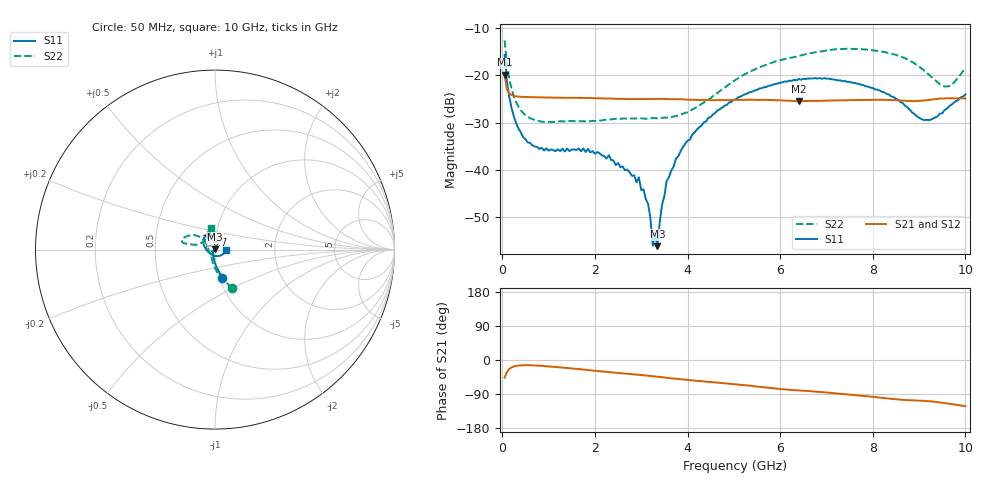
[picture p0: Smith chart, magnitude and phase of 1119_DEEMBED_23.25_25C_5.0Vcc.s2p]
!Hittite Microwave Corp.
!Digital Attenuator/PhaseShifter Rev 1.4.0
!Filename: C:\DATA\DATA\1119_DEEMBED_23.25_25C_5.0Vcc.s2p
!VNA ID: Agilent Technologies,N5224A,MY51441122,A.10.45.03
!Device type:
!2 Port Calibration.
!Temp(C): 25
!Lot Number:
!Serial Number:
!Operator:
!Misc:
!Attenuator:  23.250
# GHZ S DB R 50.0
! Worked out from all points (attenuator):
!   200 points, 50 MHz to 10 GHz, reference 50 ohm
!   highest |S21| = -19.82 dB at 50 MHz (marker M1); lowest = -25.4 dB at 6.4 GHz (marker M2)
!   lowest |S11| = -56.1 dB at 3.35 GHz (marker M3), VSWR 1.00, Z = 50 + j0.157 ohm
!   |S11| at or under -10 dB: start of sweep to end of sweep
!   |S22| runs from -29.8 to -12.6 dB; largest |S21 - S12| = 0.0002
!   S11 on the Smith chart (normalised r, x): 50 MHz: 1.03, -0.34; 6.7 GHz: 0.90, +0.15; 10 GHz: 1.13, -0.01
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0.05  -15.67 -75.6  -19.82 -46.3  -19.82 -46.3  -12.60 -66.7
0.1  -21.23 -87.8  -22.93 -31.9  -22.93 -31.9  -17.55 -83.5
0.2  -26.88 -99.9  -24.14 -19.6  -24.14 -19.6  -22.83 -100.2
0.45  -33.03 -118.1  -24.53 -13.8  -24.53 -13.8  -27.92 -120.8
0.9  -35.87 -137.8  -24.65 -15.9  -24.65 -15.9  -29.82 -135.1
1.75  -35.41 -145.1  -24.75 -25.2  -24.74 -25.2  -29.67 -139.9
2.95  -41.53 -127.8  -24.96 -39.0  -24.97 -39.1  -29.08 -158.8
3.15  -47.19 -125.6  -24.97 -41.4  -24.98 -41.5  -29.08 -164.9
3.25  -55.96 -151.2  -24.94 -42.8  -24.95 -42.9  -28.98 -167.6
3.3  -53.42 162.3  -24.96 -43.6  -24.96 -43.7  -29.03 -169.3
3.35  -56.08 87.0  -24.97 -44.2  -24.98 -44.3  -29.07 -170.9
3.4  -51.00 116.1  -24.96 -44.7  -24.97 -44.8  -29.01 -172.3
3.55  -42.23 84.4  -24.96 -47.0  -24.97 -47.1  -28.91 -177.7
3.9  -35.14 74.3  -25.05 -51.5  -25.06 -51.5  -28.11 168.0
4.45  -28.94 75.9  -25.22 -57.8  -25.24 -57.9  -25.09 147.4
5.05  -25.01 86.5  -25.18 -64.1  -25.20 -64.2  -20.85 139.4
6.4  -20.74 112.1  -25.44 -80.2  -25.46 -80.2  -15.90 150.5
6.7  -20.64 118.7  -25.37 -82.8  -25.38 -82.8  -15.20 154.5
8.35  -24.02 162.4  -25.18 -101.7  -25.18 -101.7  -15.26 168.2
9.1  -29.45 -128.8  -25.30 -107.7  -25.31 -107.8  -18.88 166.3
9.6  -27.01 -47.6  -24.84 -114.7  -24.85 -114.7  -22.34 133.4
10  -24.03 -2.0  -24.87 -121.9  -24.87 -121.9  -18.41 99.7
